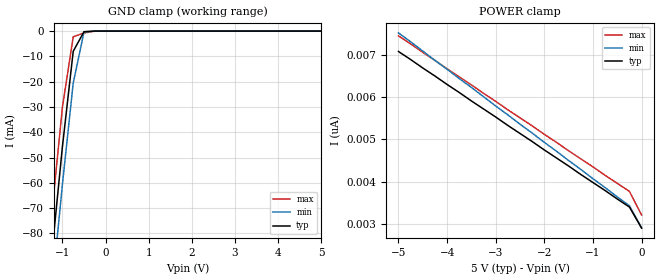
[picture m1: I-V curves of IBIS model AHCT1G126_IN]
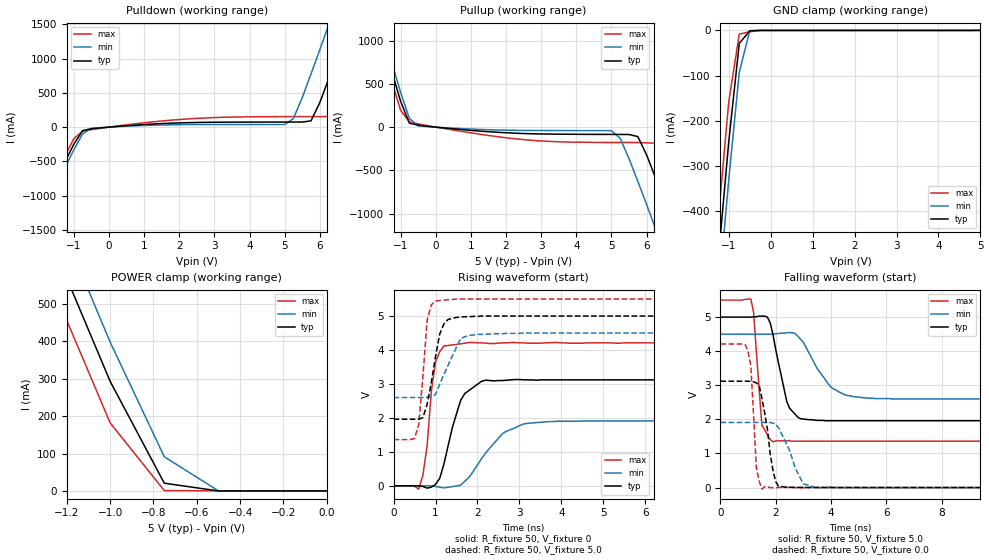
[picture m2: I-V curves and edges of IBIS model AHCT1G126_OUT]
| TEXAS INSTRUMENTS INCORPORATED
| Standard Linear and Logic Group
| IBIS Model of SN74AHCT1G126
| SINGLE BUS BUFFER GATE WITH 3-STATE OUTPUTS
| SOT 5-pin (DCK) and SOT 5-pin (DBV) Package
[IBIS Ver]   3.2
[Comment Char]  |_char
[File Name]   ahct1g126.ibs
[File Rev]   2.0 H_die
[Date]   May 24, 2000
[Source]   Data created from HSPICE simulations at TI-SLL.
[Notes]   The following is an IBIS list for the AHCT1G126.
|   Please contact sllibis@ti.com with questions and
|   comments concerning SLL IBIS models.
[Disclaimer] Property of Texas Instruments Incorporated.  Unauthorized
   reproduction and/or distribution is strictly prohibited.
   This product is protected under copyright law.
   Created 2000, (C) Copyright 2000, Texas Instruments Inc.,
   All Rights Reserved.
   UNLESS THERE IS A SIGNED, WRITTEN AGREEMENT TO THE
   CONTRARY, TEXAS INSTRUMENTS () IS PROVIDING THE IBIS
   MODELS  AND WITHOUT ANY WARRANTY, EXPRESSED OR
   IMPLIED.  TI assumes no liability for:
   1) the accuracy of the IBIS models provided to your
   company;
   2) the proper functioning of these IBIS Models in your
   design or for any resulting applications; or
   3) infringement of patents, copyrights or intellectual
   property rights resulting from your use of these IBIS
   models.
   TI provides IBIS Models as a service to our customers.
   You and your company shall not distribute, sell or give
   these models to anyone else without prior written
   permission from TI.
   TI reserves the right to make changes to our products or
   to discontinue any semiconductor product or service
   without notice, and advises our customers to obtain the
   latest version of relevant information to verify, before
   placing orders, that the information being relied on is
   current.
   Please be aware that your receipt and use of the IBIS
   information provided shall serve as acceptance of these
   terms and conditions.  If you do not accept these terms,
   you should return or destroy the IBIS models and any
   other accompanying information immediately.
|   Component AHCT1G126_DCK
[Component]   AHCT1G126_DCK
[Manufacturer]  Texas Instruments, Inc.
[Package]
|   typ   min   max
R_pkg   0.020   0.017   0.025
L_pkg   0.998nH   0.881nH   1.069nH
C_pkg   0.146pF   0.118pF   0.205pF
[Pin]   signal_name   model_name   R_pin   L_pin   C_pin
1   OE   AHCT1G126_IN   0.019   1.069nH   0.162pF
2   A   AHCT1G126_IN   0.018   0.881nH   0.121pF
3   GND   GND   0.017   1.031nH   0.205pF
4   Y   AHCT1G126_OUT   0.020   0.960nH   0.124pF
5   VCC   POWER   0.025   1.049nH   0.118pF
|   Component AHCT1G126_DBV
[Component]   AHCT1G126_DBV
[Manufacturer]  Texas Instruments, Inc.
[Package]
|   typ   min   max
R_pkg   0.025   0.021   0.029
L_pkg   1.529nH   1.312nH   1.906nH
C_pkg   0.156pF   0.110pF   0.240pF
[Pin]   signal_name   model_name   R_pin   L_pin   C_pin
1   OE   AHCT1G126_IN   0.021   1.511nH   0.144pF
2   A   AHCT1G126_IN   0.023   1.312nH   0.138pF
3   GND   GND   0.029   1.906nH   0.240pF
4   Y   AHCT1G126_OUT   0.026   1.541nH   0.150pF
5   VCC   POWER   0.025   1.374nH   0.110pF
| Models and submodels in the file (2): AHCT1G126_IN (Input), AHCT1G126_OUT (3-state)
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|   Model AHCT1G126_IN
[Model]   AHCT1G126_IN
Model_type  Input
Polarity   Inverting
Vinl = 0.8
Vinh = 2.0
| variable   typ   min   max
C_comp   1.16pf   0.87pf   1.45pf
[Temperature Range]   25   85   -40
[Voltage Range]   5.0   4.5   5.5
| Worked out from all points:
|   GND clamp passes 1 mA (typ) near -0.52 V on its own axis
[GND Clamp]
|   Voltage   I(typ)   I(min)   I(max)
-5V       -773mA     -786mA     -758mA
-1.5V     -133mA     -148mA     -117mA
-1.25V    -88.7mA    -104mA     -72.7mA
-1V       -45.6mA    -60.5mA    -30mA
-750mV    -7.99mA    -20.5mA    -2.23mA
-500mV    -233uA     -353uA     -759uA
-250mV    -2.63nA    -182nA     -26.9uA
5V        2.9nA      3.64nA     2.54nA
[POWER Clamp]
|   Voltage   I(typ)   I(min)   I(max)
-5V       7.08nA     7.52nA     7.45nA
-1.5V     4.37nA     4.5nA      4.73nA
-250mV    3.4nA      3.43nA     3.77nA
0V        2.9nA      2.91nA     3.21nA
|   Model AHCT1G126_OUT
[Model]   AHCT1G126_OUT
Model_type  3-state
Polarity   Non-Inverting
Enable   Active-High
Vmeas = 2.5v
Cref = 15pf
| variable   typ   min   max
C_comp   4.1pf   3.075pf   5.125pf
[Temperature Range]   25   85   -40
[Voltage Range]   5.0   4.5   5.5
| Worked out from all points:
|   slope of the pulldown table from 0 to 0.75 V, typ, clamps not added: 24.8 ohm
|   slope of the pullup table from 0 to 0.75 V, typ, clamps not added: 25.9 ohm
|   GND clamp passes 1 mA (typ) near -0.50 V on its own axis
|   POWER clamp passes 1 mA (typ) near -0.51 V on its own axis
|   rising waveform, R_fixture 50, V_fixture 0: 20-80 % time 398ps typ, 717ps min, 208ps max; typ from 0 V to 3.12 V
|   falling waveform, R_fixture 50, V_fixture 5.0: 20-80 % time 465ps typ, 867ps min, 226ps max; typ from 5 V to 1.96 V
|   rising waveform, R_fixture 50, V_fixture 5.0: 20-80 % time 262ps typ, 419ps min, 161ps max; typ from 1.96 V to 5 V
|   falling waveform, R_fixture 50, V_fixture 0.0: 20-80 % time 346ps typ, 585ps min, 169ps max; typ from 3.12 V to 0 V
[Pulldown]
|   Voltage   I(typ)   I(min)   I(max)
-5V       -4.66A     -4.73A     -4.58A
-2.25V    -1.6A      -1.68A     -1.51A
-2V       -1.32A     -1.4A      -1.23A
-1V       -250mA     -331mA     -170mA
-500mV    -23.5mA    -16.1mA    -37.4mA
5V        74.6mA     38.5mA     154mA
5.75V     91.7mA     776mA      154mA
6.25V     701mA      1.49A      155mA
6.75V     1.42A      2.22A      657mA
7.25V     2.15A      2.96A      1.38A
7.5V      2.52A      3.33A      1.75A
10V       6.23A      7.04A      5.45A
[Pullup]
|   Voltage   I(typ)   I(min)   I(max)
-5V       6.17A      6.26A      6.07A
-1.75V    1.36A      1.46A      1.25A
-1.5V     996mA      1.1A       886mA
-1V       298mA      400mA      194mA
-750mV    45.7mA     98.7mA     59.2mA
-500mV    23mA       14.9mA     37.9mA
5V        -84.3mA    -40.9mA    -178mA
5.75V     -109mA     -626mA     -178mA
6.25V     -581mA     -1.17A     -186mA
6.75V     -1.12A     -1.71A     -574mA
7.25V     -1.67A     -2.27A     -1.12A
10V       -4.73A     -5.33A     -4.18A
[GND Clamp]
|   Voltage   I(typ)   I(min)   I(max)
-5V       -4.66A     -4.73A     -4.58A
-1.5V     -774mA     -858mA     -684mA
-1.25V    -505mA     -590mA     -415mA
-1V       -245mA     -329mA     -157mA
-750mV    -28.8mA    -92.4mA    -8.32mA
-500mV    -878uA     -589uA     -2.99mA
-250mV    -21.8nA    -122nA     -114uA
5V        2nA        199uA      1.9nA
[POWER Clamp]
|   Voltage   I(typ)   I(min)   I(max)
-5V       6.17A      6.26A      6.07A
-1.25V    637mA      743mA      524mA
-1V       293mA      398mA      182mA
-750mV    20.6mA     91.3mA     1.05mA
-500mV    2.09uA     199uA      42uA
0V        2nA        1.97nA     2.2nA
[Ramp]
| variable   typ   min   max
dV/dt_r   1.89E+00/4.14E-10   1.15E+00/7.26E-10   2.52E+00/1.91E-10
dV/dt_f   1.85E+00/4.80E-10   1.17E+00/9.02E-10   2.24E+00/2.50E-10
R_load = 50
[Rising Waveform]
R_fixture = 50
V_fixture = 0
|   Time   V(typ)   V(min)   V(max)
0s        0V         0V         0V
600ps     -498uV     230uV      -99.9mV
800ps     -68.6mV    -69.7uV    1.19V
1ns       41.1mV     -20mV      3.65V
1.2ns     640mV      -62.6mV    4.12V
1.6ns     2.52V      16.9mV     4.18V
2.2ns     3.11V      975mV      4.2V
2.7ns     3.11V      1.61V      4.21V
3.9ns     3.12V      1.9V       4.22V
25ns      3.12V      1.91V      4.21V
[Falling Waveform]
R_fixture = 50
V_fixture = 5.0
V_fixture_min = 4.5
V_fixture_max = 5.5
|   Time   V(typ)   V(min)   V(max)
0s        5V         4.5V       5.5V
1.1ns     5V         4.5V       5.53V
1.2ns     5.01V      4.5V       5.14V
1.5ns     5.03V      4.5V       1.83V
1.9ns     4.49V      4.5V       1.34V
2.4ns     2.52V      4.54V      1.37V
2.9ns     2.02V      4.35V      1.36V
4ns       1.96V      2.94V      1.36V
5.2ns     1.96V      2.63V      1.36V
25ns      1.96V      2.6V       1.36V
[Rising Waveform]
R_fixture = 50
V_fixture = 5.0
V_fixture_min = 4.5
V_fixture_max = 5.5
|   Time   V(typ)   V(min)   V(max)
0s        1.96V      2.6V       1.36V
500ps     1.96V      2.6V       1.39V
600ps     1.96V      2.6V       1.81V
800ps     2.4V       2.61V      4.88V
900ps     3.05V      2.62V      5.33V
1.1ns     4.47V      2.99V      5.46V
1.3ns     4.9V       3.55V      5.48V
1.6ns     4.97V      4.34V      5.5V
2ns       4.99V      4.46V      5.5V
25ns      5V         4.5V       5.5V
[Falling Waveform]
R_fixture = 50
V_fixture = 0.0
|   Time   V(typ)   V(min)   V(max)
0s        3.12V      1.91V      4.21V
1ns       3.12V      1.91V      3.99V
1.1ns     3.11V      1.91V      3.57V
1.3ns     3.07V      1.91V      572mV
1.5ns     2.62V      1.91V      -47.6mV
2ns       172mV      1.86V      -923uV
2.3ns     16.3mV     1.43V      5.99mV
3ns       1.88mV     108mV      -966uV
3.5ns     493uV      -4.71mV    904uV
25ns      0V         0V         0V
